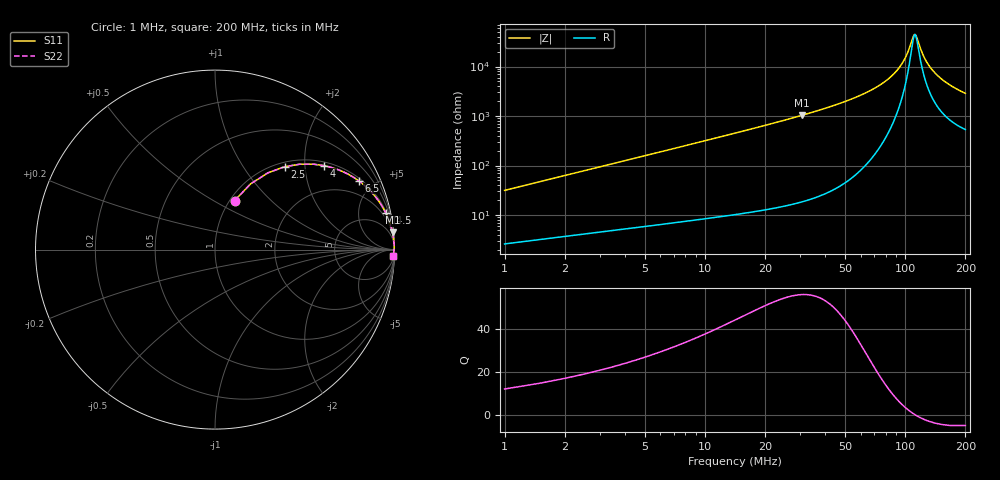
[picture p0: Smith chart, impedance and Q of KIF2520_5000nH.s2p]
!version-2
!date-12.2020
!Series
# MHz S RI R 50
!Freq ReS11 ImS11 ReS21 ImS21 ReS12 ImS12 ReS22 ImS22
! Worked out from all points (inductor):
!   399 points, 1 MHz to 200 MHz, reference 50 ohm
!   read as one part in series: L = 5 uH near 1.5 MHz
!   highest Q = 56.1 at 30.5 MHz (marker M1), where L = 5.4 uH
!   self-resonance near 112 MHz
!   S11 on the Smith chart (normalised r, x): 1 MHz: 1.05, +0.63; 2.5 MHz: 1.08, +1.57; 4 MHz: 1.10, +2.52; 6.5 MHz: 1.13, +4.10; 14.5 MHz: 1.21, +9.27; 200 MHz: 12, -57
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1  0.109 0.2728  0.891 -0.2728  0.891 -0.2728  0.109 0.2728
1.5  0.1982 0.3662  0.8018 -0.3662  0.8018 -0.3662  0.1982 0.3662
2.5  0.3881 0.4617  0.6119 -0.4617  0.6119 -0.4617  0.3881 0.4617
4  0.6089 0.4676  0.3911 -0.4676  0.3911 -0.4676  0.6089 0.4676
6.5  0.8001 0.3839  0.1999 -0.3839  0.1999 -0.3839  0.8001 0.3839
9.5  0.894 0.2945  0.106 -0.2945  0.106 -0.2945  0.894 0.2945
14.5  0.9513 0.2042  0.0487 -0.2042  0.0487 -0.2042  0.9513 0.2042
21.5  0.9775 0.139  0.0225 -0.139  0.0225 -0.139  0.9775 0.139
30.5  0.9891 0.0954  0.0109 -0.0954  0.0109 -0.0954  0.9891 0.0954
34.5  0.9916 0.0826  0.00838 -0.0826  0.00838 -0.0826  0.9916 0.0826
67.5  0.9979 0.0299  0.00211 -0.0299  0.00211 -0.0299  0.9979 0.0299
87.5  0.9982 0.0141  0.00176 -0.0141  0.00176 -0.0141  0.9982 0.0141
94.5  0.9982 0.00969  0.00182 -0.00969  0.00182 -0.00969  0.9982 0.00969
100.5  0.9981 0.00618  0.00193 -0.00618  0.00193 -0.00618  0.9981 0.00618
109.5  0.9978 0.00133  0.00216 -0.00133  0.00216 -0.00133  0.9978 0.00133
112  0.9978 6.19e-05  0.00224 -6.19e-05  0.00224 -6.19e-05  0.9978 6.19e-05
114  0.9977 -0.000933  0.00231 0.000933  0.00231 0.000933  0.9977 -0.000933
123.5  0.9973 -0.00543  0.00267 0.00543  0.00267 0.00543  0.9973 -0.00543
134  0.9969 -0.01  0.00315 0.01  0.00315 0.01  0.9969 -0.01
148  0.9961 -0.0157  0.0039 0.0157  0.0039 0.0157  0.9961 -0.0157
167  0.9949 -0.0227  0.00509 0.0227  0.00509 0.0227  0.9949 -0.0227
200  0.9924 -0.0337  0.00757 0.0337  0.00757 0.0337  0.9924 -0.0337
